| IBIS file stm32u073_083_lqfp64.ibs
[IBIS ver] 4.2
[File name] stm32u073_083_lqfp64.ibs
[File Rev] 0.3
[Date] 20-02-2024
[Source] Data Created at STMicroelectronics
[Notes]  File originated from ELDO simulations.
[Disclaimer]  This information is for modeling purpose only and is
   not guaranteed. The information is subject to change without
   notice.
[Copyright] Copyright 2024 STMicroelectronics Inc.
|   Component stm32u073_083_lqfp64
[Component] stm32u073_083_lqfp64
[Manufacturer] STMicroelectronics
[Package]
| variable   typ   min   max
R_pkg  0  NA  NA
L_pkg  0  NA  NA
C_pkg  0  NA  NA
[Pin]   signal_name   model_name
1  VBAT  power
2  PC13  io8_ft_v33
3  PC14-OSC32_IN  io8_ft_v33
4  PC15-OSC32_OUT  io8_ft
5  PF0-OSC_IN  io8_ft
6  PF1-OSC_OUT  io8_ft
7  PF2-NRST  ioreset_ft_v33
8  PC0  io8_ft_i2c
9  PC1  io8_ft_i2c
10  PC2  io8_ft
11  PC3  io8_ft
12  VSSA_VREFM  nc
13  VDDA_VREFP  nc
14  PA0  io8_ft_v33
15  PA1  io8_ft_v33
16  PA2  io8_ft_v33
17  PA3  io8_ft
18  VSS  gnd
19  VDD  power
20  PA4  io8_ft
21  PA5  io8_ft
22  PA6  io8_ft_i2c
23  PA7  io8_ft_i2c
24  PC4  io8_ft
25  PC5  io8_ft_v33
26  PB0  io8_ft
27  PB1  io8_ft
28  PB2  io8_ft
29  PB10  io8_ft_i2c
30  PB11  io8_ft_i2c
31  VSS  gnd
32  VDD  power
33  PB12  io8_ft
34  PB13  io8_ft_i2c
35  PB14  io8_ft_i2c
36  PB15  io8_ft_v33
37  PC6  io8_ft
38  PC7  io8_ft
39  PC8  io8_ft
40  PC9  io8_ft
41  PA8  io8_ft
42  PA9  io8_ft_i2c
43  PA10  io8_ft_i2c
44  PA11  io8usb_ft_phy
45  PA12  io8usb_ft_phy
46  PA13  io8_ft
47  VSS  gnd
48  VDDUSB  power
49  PA14  io8_ft
50  PA15  io8_ft
51  PC10  io8_ft
52  PC11  io8_ft
53  PC12  io8_ft
54  PD2  io8_ft
55  PB3  io8_ft_i2c
56  PB4  io8_ft_i2c
57  PB5  io8_ft
58  PB6  io8_ft_i2c
59  PB7  io8_ft_i2c
60  PF3-BOOT0  io8_ft_v33
61  PB8  io8_ft_i2c
62  PB9  io8_ft_i2c
63  VSS  gnd
64  VDD  power
[Package Model]   489-lqfp-10x10-64-ldo-240126
[Pin Mapping]   pulldown_ref   pullup_ref   | Comment
1  nc  vsw
2  gndio  vddio  | Depending on IO usage
| 2  gndio  vsw  | Depending on IO usage
3  gndio  vddio  | Depending on IO usage
| 3  gndio  vsw  | Depending on IO usage
4  gndio  vddio  | Depending on IO usage
| 4  gndio  vsw  | Depending on IO usage
5  gndio  vddio
6  gndio  vddio
7  gndio  vddio
8  gndio  vddio
9  gndio  vddio
10  gndio  vddio
11  gndio  vddio
12  nc  nc
13  nc  nc
14  gndio  vddio
15  gndio  vddio
16  gndio  vddio
17  gndio  vddio
18  gndio  nc
19  nc  vddio
20  gndio  vddio
21  gndio  vddio
22  gndio  vddio
23  gndio  vddio
24  gndio  vddio
25  gndio  vddio
26  gndio  vddio
27  gndio  vddio
28  gndio  vddio
29  gndio  vddio
30  gndio  vddio
31  gndio  nc
32  nc  vddio
33  gndio  vddio
34  gndio  vddio
35  gndio  vddio
36  gndio  vddio
37  gndio  vddio
38  gndio  vddio
39  gndio  vddio
40  gndio  vddio
41  gndio  vddio
42  gndio  vddio
43  gndio  vddio
44  gndio  vddusb  | Depending on IO usage
| 44  gndio  vddio  | Depending on IO usage
45  gndio  vddusb  | Depending on IO usage
| 45  gndio  vddio  | Depending on IO usage
46  gndio  vddio
47  gndio  nc
48  nc  vddusb
49  gndio  vddio
50  gndio  vddio
51  gndio  vddio
52  gndio  vddio
53  gndio  vddio
54  gndio  vddio
55  gndio  vddio
56  gndio  vddio
57  gndio  vddio
58  gndio  vddio
59  gndio  vddio
60  gndio  vddio
61  gndio  vddio
62  gndio  vddio
63  gndio  nc
64  nc  vddio
|[Diff Pin]  inv_pin  vdiff  tdelay_typ  tdelay_min  tdelay_max
|45  44  NA  NA  NA  NA
[Model Selector] io8_ft
io8_ft_ls_1v2   "GPIO - 5V tolerant - 1.2V range - Low speed"
io8_ft_ms_1v2   "GPIO - 5V tolerant - 1.2V range - Med speed"
io8_ft_fs_1v2   "GPIO - 5V tolerant - 1.2V range - Fast speed"
io8_ft_hs_1v2   "GPIO - 5V tolerant - 1.2V range - High speed"
io8_ft_ls_1v8   "GPIO - 5V tolerant - 1.8V range - Low speed"
io8_ft_ms_1v8   "GPIO - 5V tolerant - 1.8V range - Med speed"
io8_ft_fs_1v8   "GPIO - 5V tolerant - 1.8V range - Fast speed"
io8_ft_hs_1v8   "GPIO - 5V tolerant - 1.8V range - High speed"
io8_ft_ls_3v3   "GPIO - 5V tolerant - 3.3V range - Low speed"
io8_ft_ms_3v3   "GPIO - 5V tolerant - 3.3V range - Med speed"
io8_ft_fs_3v3   "GPIO - 5V tolerant - 3.3V range - Fast speed"
io8_ft_hs_3v3   "GPIO - 5V tolerant - 3.3V range - High speed"
[Model Selector] io8_ft_i2c
io8_ft_ls_1v2   "GPIO - 5V tolerant - 1.2V range - Low speed"
io8_ft_ms_1v2   "GPIO - 5V tolerant - 1.2V range - Med speed"
io8_ft_fs_1v2   "GPIO - 5V tolerant - 1.2V range - Fast speed"
io8_ft_hs_1v2   "GPIO - 5V tolerant - 1.2V range - High speed"
io8_ft_ls_1v8   "GPIO - 5V tolerant - 1.8V range - Low speed"
io8_ft_ms_1v8   "GPIO - 5V tolerant - 1.8V range - Med speed"
io8_ft_fs_1v8   "GPIO - 5V tolerant - 1.8V range - Fast speed"
io8_ft_hs_1v8   "GPIO - 5V tolerant - 1.8V range - High speed"
io8_ft_ls_3v3   "GPIO - 5V tolerant - 3.3V range - Low speed"
io8_ft_ms_3v3   "GPIO - 5V tolerant - 3.3V range - Med speed"
io8_ft_fs_3v3   "GPIO - 5V tolerant - 3.3V range - Fast speed"
io8_ft_hs_3v3   "GPIO - 5V tolerant - 3.3V range - High speed"
io8_ft_i2c_ls_1v2   "GPIO I2C open-drain - 5V tolerant - 1.2V range - Low speed"
io8_ft_i2c_ms_1v2   "GPIO I2C open-drain - 5V tolerant - 1.2V range - Med speed"
io8_ft_i2c_fs_1v2   "GPIO I2C open-drain - 5V tolerant - 1.2V range - Fast speed"
io8_ft_i2c_hs_1v2   "GPIO I2C open-drain - 5V tolerant - 1.2V range - High speed"
io8_ft_i2c_ls_1v8   "GPIO I2C open-drain - 5V tolerant - 1.8V range - Low speed"
io8_ft_i2c_ms_1v8   "GPIO I2C open-drain - 5V tolerant - 1.8V range - Med speed"
io8_ft_i2c_fs_1v8   "GPIO I2C open-drain - 5V tolerant - 1.8V range - Fast speed"
io8_ft_i2c_hs_1v8   "GPIO I2C open-drain - 5V tolerant - 1.8V range - High speed"
io8_ft_i2c_ls_3v3   "GPIO I2C open-drain - 5V tolerant - 3.3V range - Low speed"
io8_ft_i2c_ms_3v3   "GPIO I2C open-drain - 5V tolerant - 3.3V range - Med speed"
io8_ft_i2c_fs_3v3   "GPIO I2C open-drain - 5V tolerant - 3.3V range - Fast speed"
io8_ft_i2c_hs_3v3   "GPIO I2C open-drain - 5V tolerant - 3.3V range - High speed"
io8_ft_i2c_fmp_3v3   "GPIO I2C open-drain fm+ - 5V tolerant - 3.3V range"
[Model Selector] io8_ft_v33
io8_ft_v33_ls_1v2   "GPIO_V33 - 5V tolerant - 1.2V range - Low speed"
io8_ft_v33_ms_1v2   "GPIO_V33 - 5V tolerant - 1.2V range - Med speed"
io8_ft_v33_fs_1v2   "GPIO_V33 - 5V tolerant - 1.2V range - Fast speed"
io8_ft_v33_hs_1v2   "GPIO_V33 - 5V tolerant - 1.2V range - High speed"
io8_ft_v33_ls_1v8   "GPIO_V33 - 5V tolerant - 1.8V range - Low speed"
io8_ft_v33_ms_1v8   "GPIO_V33 - 5V tolerant - 1.8V range - Med speed"
io8_ft_v33_fs_1v8   "GPIO_V33 - 5V tolerant - 1.8V range - Fast speed"
io8_ft_v33_hs_1v8   "GPIO_V33 - 5V tolerant - 1.8V range - High speed"
io8_ft_v33_ls_3v3   "GPIO_V33 - 5V tolerant - 3.3V range - Low speed"
io8_ft_v33_ms_3v3   "GPIO_V33 - 5V tolerant - 3.3V range - Med speed"
io8_ft_v33_fs_3v3   "GPIO_V33 - 5V tolerant - 3.3V range - Fast speed"
io8_ft_v33_hs_3v3   "GPIO_V33 - 5V tolerant - 3.3V range - High speed"
[Model Selector] io8usb_ft_phy
io8_ft_ls_1v2   "GPIO - 5V tolerant - 1.2V range - Low speed"
io8_ft_ms_1v2   "GPIO - 5V tolerant - 1.2V range - Med speed"
io8_ft_fs_1v2   "GPIO - 5V tolerant - 1.2V range - Fast speed"
io8_ft_hs_1v2   "GPIO - 5V tolerant - 1.2V range - High speed"
io8_ft_ls_1v8   "GPIO - 5V tolerant - 1.8V range - Low speed"
io8_ft_ms_1v8   "GPIO - 5V tolerant - 1.8V range - Med speed"
io8_ft_fs_1v8   "GPIO - 5V tolerant - 1.8V range - Fast speed"
io8_ft_hs_1v8   "GPIO - 5V tolerant - 1.8V range - High speed"
io8_ft_ls_3v3   "GPIO - 5V tolerant - 3.3V range - Low speed"
io8_ft_ms_3v3   "GPIO - 5V tolerant - 3.3V range - Med speed"
io8_ft_fs_3v3   "GPIO - 5V tolerant - 3.3V range - Fast speed"
io8_ft_hs_3v3   "GPIO - 5V tolerant - 3.3V range - High speed"
io8usb_ft_phy_hs_3v3   "USB full speed"
io8usb_ft_phy_ls_3v3   "USB low speed"
[Model Selector] ioreset_ft_v33
ioreset_ft_v33_1v2   "Reset PAD. 5V tolerant. 1.2V range"
ioreset_ft_v33_1v8   "Reset PAD. 5V tolerant. 1.8V range"
ioreset_ft_v33_3v3   "Reset PAD. 5V tolerant. 3.3V range"
[Define Package Model]  489-lqfp-10x10-64-ldo-240126
[Manufacturer]  Unknown
[OEM]  Unknown
[Description]  None
[Number Of Pins]  61
[Pin Numbers]
| Pin Num   Terminal Name
14 | PA0
15 | PA1
16 | PA2
17 | PA3
20 | PA4
21 | PA5
22 | PA6
23 | PA7
41 | PA8
42 | PA9
43 | PA10
44 | PA11
45 | PA12
46 | PA13
49 | PA14
50 | PA15
26 | PB0
27 | PB1
28 | PB2
55 | PB3
56 | PB4
57 | PB5
58 | PB6
59 | PB7
61 | PB8
62 | PB9
29 | PB10
30 | PB11
33 | PB12
34 | PB13
35 | PB14
36 | PB15
8 | PC0
9 | PC1
10 | PC2
11 | PC3
24 | PC4
25 | PC5
37 | PC6
38 | PC7
39 | PC8
40 | PC9
51 | PC10
52 | PC11
53 | PC12
2 | PC13
3 | PC14-OSC32_IN
4 | PC15-OSC32_OUT
54 | PD2
60 | PF3-BOOT0
5 | PF0-OSC_IN
6 | PF1-OSC_OUT
7 | PF2-NRST
1 | VBAT
64 | VDD
19 | VDD
32 | VDD
13 | VDDA_VREFP
48 | VDDUSB
18 | VSS
12 | VSSA_VREFM
|[Merged Pins]  18
|31  |  VSS
|47  |  VSS
|63  |  VSS
[Model Data]
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[End Model Data]
[End Package Model]
|End [Component]
| Models and submodels in the file (42): io8_ft_fs_1v2 (I/O), io8_ft_fs_1v8 (I/O), io8_ft_fs_3v3 (I/O), io8_ft_hs_1v2 (I/O), io8_ft_hs_1v8 (I/O), io8_ft_hs_3v3 (I/O), io8_ft_i2c_fmp_3v3 (I/O_open_drain), io8_ft_i2c_fs_1v2 (I/O_open_drain), io8_ft_i2c_fs_1v8 (I/O_open_drain), io8_ft_i2c_fs_3v3 (I/O_open_drain), io8_ft_i2c_hs_1v2 (I/O_open_drain), io8_ft_i2c_hs_1v8 (I/O_open_drain), io8_ft_i2c_hs_3v3 (I/O_open_drain), io8_ft_i2c_ls_1v2 (I/O_open_drain), io8_ft_i2c_ls_1v8 (I/O_open_drain), io8_ft_i2c_ls_3v3 (I/O_open_drain), io8_ft_i2c_ms_1v2 (I/O_open_drain), io8_ft_i2c_ms_1v8 (I/O_open_drain), io8_ft_i2c_ms_3v3 (I/O_open_drain), io8_ft_ls_1v2 (I/O), io8_ft_ls_1v8 (I/O), io8_ft_ls_3v3 (I/O), io8_ft_ms_1v2 (I/O), io8_ft_ms_1v8 (I/O), io8_ft_ms_3v3 (I/O), io8_ft_v33_fs_1v2 (I/O), io8_ft_v33_fs_1v8 (I/O), io8_ft_v33_fs_3v3 (I/O), io8_ft_v33_hs_1v2 (I/O), io8_ft_v33_hs_1v8 (I/O), io8_ft_v33_hs_3v3 (I/O), io8_ft_v33_ls_1v2 (I/O), io8_ft_v33_ls_1v8 (I/O), io8_ft_v33_ls_3v3 (I/O), io8_ft_v33_ms_1v2 (I/O), io8_ft_v33_ms_1v8 (I/O), io8_ft_v33_ms_3v3 (I/O), io8usb_ft_phy_hs_3v3 (I/O), io8usb_ft_phy_ls_3v3 (I/O), ioreset_ft_v33_1v2 (I/O_open_drain), ioreset_ft_v33_1v8 (I/O_open_drain), ioreset_ft_v33_3v3 (I/O_open_drain)
